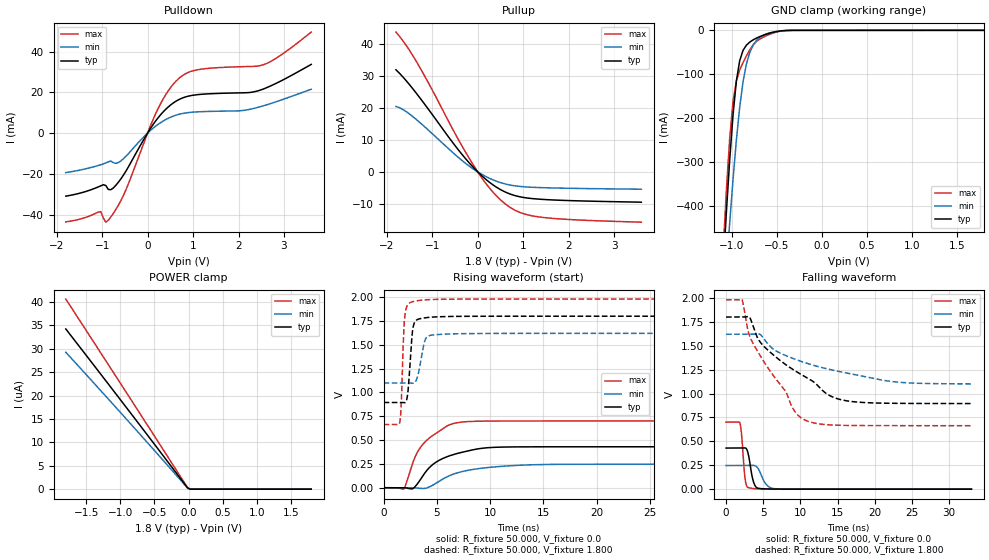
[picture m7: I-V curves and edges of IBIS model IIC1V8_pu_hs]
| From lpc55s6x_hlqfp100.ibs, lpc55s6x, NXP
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|   Model IIC1V8_pu_hs
[Model] IIC1V8_pu_hs
Model_type I/O
Polarity   Non-Inverting
Enable   Active-Low
Vinl =  0.540V
Vinh =  1.260V
Vmeas =  0.900V
Cref =  0.0F
Rref =  100.000
Vref =  0.0V
C_comp   2.515pF   2.512pF   2.536pF
C_comp_pullup   0.457pF   0.390pF   0.548pF
C_comp_pulldown   1.734pF   1.669pF   1.790pF
[Model Spec]
Vinh   1.260V   1.134V   1.386V
Vinl   0.540V   0.486V   0.594V
Vmeas   0.900V   0.810V   0.990V
Vref   0.0V   0.0V   0.0V
Cref   0.0F   0.0F   0.0F
Rref   1000.000   1000.000   1000.000
[Temperature Range]   25.000   0.125k   -40.000
[Voltage Range]   1.800V   1.620V   1.980V
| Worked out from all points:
|   slope of the pulldown table from 0 to 0.27 V, typ, clamps not added: 31.5 ohm
|   slope of the pullup table from 0 to 0.27 V, typ, clamps not added: 79.6 ohm
|   GND clamp passes 1 mA (typ) near -0.44 V on its own axis
|   rising waveform, R_fixture 50.000, V_fixture 0.0: 20-80 % time 2.97ns typ, 3.77ns min, 2.39ns max; typ from 0.001 V to 0.43 V
|   rising waveform, R_fixture 50.000, V_fixture 1.800: 20-80 % time 347ps typ, 536ps min, 254ps max; typ from 0.895 V to 1.8 V
|   falling waveform, R_fixture 50.000, V_fixture 0.0: 20-80 % time 599ps typ, 965ps min, 410ps max; typ from 0.43 V to 0.001 V
|   falling waveform, R_fixture 50.000, V_fixture 1.800: 20-80 % time 8.38ns typ, 11.2ns min, 5.71ns max; typ from 1.8 V to 0.896 V
[Pulldown]
|Voltage   I(typ)   I(min)   I(max)
-1.8V     -30.97mA   -19.41mA   -43.61mA
-1.03V    -25.91mA   -15.56mA   -38.59mA
-920mV    -25.75mA   -14.67mA   -43.75mA
-865mV    -27.69mA   -14.16mA   -42.79mA
-700mV    -25.69mA   -14.87mA   -37.58mA
-480mV    -18.8mA    -11.48mA   -28.03mA
235mV     7.619mA    4.356mA    12.23mA
455mV     12.83mA    7.267mA    20.76mA
730mV     16.88mA    9.427mA    27.6mA
1.17V     19mA       10.49mA    31.33mA
2.545V    21.61mA    13.36mA    33.53mA
3.6V      33.71mA    21.52mA    49.57mA
[Pullup]
|Voltage   I(typ)   I(min)   I(max)
-1.8V     32.05mA    20.54mA    43.88mA
-1.57V    28.56mA    18.87mA    39.61mA
-1.295V   23.65mA    15.77mA    33.3mA
-1.02V    18.4mA     12.24mA    26.22mA
-470mV    7.714mA    5.076mA    11.29mA
-30mV     432.2uA    271.3uA    660.2uA
300mV     -3.713mA   -2.28mA    -5.781mA
630mV     -6.475mA   -3.874mA   -10.31mA
960mV     -7.909mA   -4.606mA   -12.9mA
1.4V      -8.61mA    -4.943mA   -14.23mA
2.17V     -9.075mA   -5.188mA   -15.07mA
3.6V      -9.515mA   -5.442mA   -15.79mA
[GND_clamp]
|Voltage   I(typ)   I(min)   I(max)
-1.8V     -3.488A    -3.23A     -3.872A
-1.097V   -545.6mA   -658.5mA   -507.1mA
-1.06V    -414.6mA   -546.1mA   -365.1mA
-1.023V   -294.9mA   -439.1mA   -246mA
-986mV    -192.5mA   -339.6mA   -162mA
-949mV    -115.7mA   -250.4mA   -115.2mA
-912mV    -69.22mA   -175.3mA   -90.67mA
-838mV    -34.06mA   -77.19mA   -58.54mA
-764mV    -21.86mA   -34.13mA   -33.64mA
-653mV    -11.47mA   -11.68mA   -15.87mA
-431mV    -870uA     -906.4uA   -1.185mA
1.8V      0A         0A         0A
[POWER_clamp]
|Voltage   I(typ)   I(min)   I(max)
-1.8V     34.22uA    29.25uA    40.61uA
-864mV    16.54uA    14.2uA     19.57uA
-13mV     251.2nA    223.3nA    296.4nA
24mV      0A         0A         0A
1.8V      0A         0A         0A
[Ramp]
| variable   typ   min   max
dV/dt_r   0.258/2.973n   0.148/3.773n   0.420/2.388n
dV/dt_f   0.543/8.379n   0.311/11.175n   0.789/5.715n
R_load = 50.000
[Rising Waveform]
R_fixture= 50.000
V_fixture= 0.0
V_fixture_min= 0.0
V_fixture_max= 0.0
|time   V(typ)   V(min)   V(max)
0s        607.1uV    649.4uV    568.8uV
1.893ns   800.5uV    649.2uV    -11.6mV
2.771ns   -7.625mV   611.8uV    272.9mV
3.584ns   108.4mV    -7.321mV   442.5mV
4.864ns   264.4mV    43.55mV    567.5mV
5.944ns   325.6mV    114.7mV    647.7mV
6.834ns   357.5mV    153.6mV    681.1mV
9.469ns   417.3mV    208.6mV    699.4mV
13.65ns   429.7mV    240.3mV    700.9mV
33ns      430.3mV    247.5mV    701.1mV
[Rising Waveform]
R_fixture= 50.000
V_fixture= 1.800
V_fixture_min= 1.620
V_fixture_max= 1.980
|time   V(typ)   V(min)   V(max)
0s        895.1mV    1.1V       664.1mV
1.519ns   895.1mV    1.1V       690.2mV
1.646ns   895.3mV    1.1V       857.7mV
1.975ns   892.5mV    1.1V       1.785V
2.274ns   999mV      1.1V       1.923V
2.631ns   1.554V     1.097V     1.949V
3.003ns   1.751V     1.117V     1.959V
3.882ns   1.783V     1.547V     1.972V
4.436ns   1.79V      1.601V     1.975V
33ns      1.8V       1.62V      1.98V
[Falling Waveform]
R_fixture= 50.000
V_fixture= 0.0
V_fixture_min= 0.0
V_fixture_max= 0.0
|time   V(typ)   V(min)   V(max)
0s        430.3mV    247.6mV    701.2mV
1.861ns   430.3mV    247.6mV    693.5mV
2.09ns    430.3mV    247.6mV    569.6mV
2.556ns   432mV      247.6mV    110.6mV
3.075ns   335.2mV    247.6mV    14.74mV
3.699ns   74.36mV    248.7mV    6.459mV
4.461ns   8.322mV    196.1mV    2.834mV
5.384ns   3.28mV     52.55mV    1.435mV
6.464ns   1.643mV    6mV        892.8uV
33ns      608.1uV    651.4uV    569.3uV
[Falling Waveform]
R_fixture= 50.000
V_fixture= 1.800
V_fixture_min= 1.620
V_fixture_max= 1.980
|time   V(typ)   V(min)   V(max)
0s        1.8V       1.62V      1.98V
2.139ns   1.8V       1.62V      1.983V
2.946ns   1.806V     1.62V      1.658V
3.557ns   1.724V     1.62V      1.535V
5.14ns    1.49V      1.566V     1.328V
7.978ns   1.305V     1.399V     1.027V
9.229ns   1.24V      1.36V      814.4mV
10.51ns   1.182V     1.325V     726.9mV
16.2ns    924.3mV    1.215V     667mV
33ns      895.7mV    1.101V     664.3mV
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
